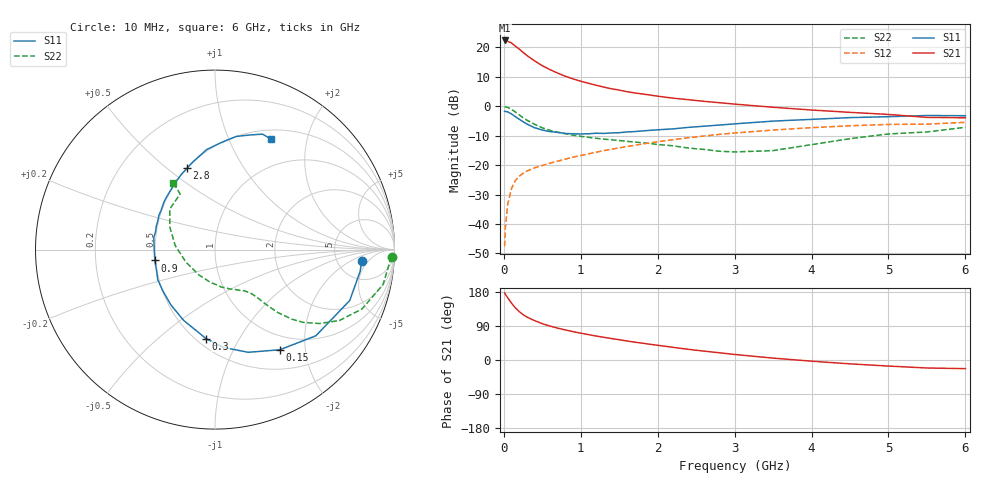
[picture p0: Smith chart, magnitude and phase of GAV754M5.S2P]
! Infineon Technologies  Discrete & RF Semiconductors
! BF775
! Si NPN RF Bipolar Junction Transistor in SOT23
! VCE = 0.75 V  IC = 4.5 mA
! Common Emitter S-Parameters:  May  1996
# GHz  S  MA  R  50
!  f  S11  S21  S12  S22
! GHz  MAG  ANG  MAG  ANG  MAG  ANG  MAG  ANG
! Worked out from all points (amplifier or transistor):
!   36 points, 10 MHz to 6 GHz, reference 50 ohm
!   highest |S21| = 22.4 dB at 10 MHz (marker M1)
!   |S21| within 3 dB of that: start of sweep to 203.1 MHz
!   unconditionally stable (mu >= 1): 727.6 MHz to end of sweep
!   at 250 MHz: K = 0.49, MSG = 20.5 dB, |S12| = -22.8 dB
!   at 1.4 GHz: K = 1.19, MAG = 7.6 dB, |S12| = -14.6 dB
!   at 6 GHz: K = 1.05, MAG = -0.6 dB, |S12| = -5.5 dB
!   S11 on the Smith chart (normalised r, x): 10 MHz: 8.86, -3.33; 150 MHz: 0.78, -1.55; 300 MHz: 0.56, -0.73; 900 MHz: 0.49, -0.07; 2.8 GHz: 0.50, +0.59; 6 GHz: 0.62, +1.45
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0.01  0.8202 -4.3  13.11 177.0  0.0042 87.2  0.9851 -2.4
0.02  0.8178 -8.5  12.94 173.5  0.0087 84.9  0.9741 -4.7
0.05  0.8025 -20.7  12.72 164.3  0.0216 78.7  0.9565 -11.7
0.1  0.7391 -40.5  11.85 150.0  0.04 69.7  0.8832 -22.0
0.15  0.6647 -57.1  10.49 137.5  0.0548 62.1  0.7977 -29.7
0.2  0.6013 -72.1  9.356 127.8  0.0645 57.0  0.7129 -35.3
0.25  0.5463 -85.3  8.24 119.7  0.0727 53.1  0.6378 -39.5
0.3  0.4981 -95.8  7.28 113.4  0.0791 51.6  0.5793 -42.1
0.4  0.4316 -113.8  5.892 103.9  0.09 49.1  0.494 -45.1
0.5  0.394 -128.7  4.88 95.8  0.0987 48.7  0.4303 -46.7
0.6  0.3704 -141.7  4.183 89.5  0.108 48.9  0.3897 -47.7
0.7  0.3604 -152.1  3.657 84.0  0.1168 49.2  0.3621 -48.4
0.9  0.3406 -169.8  2.913 74.8  0.1366 49.6  0.3229 -50.1
1.1  0.3406 175.4  2.455 67.0  0.1555 50.0  0.2964 -52.7
1.3  0.3456 163.5  2.114 59.9  0.1763 49.7  0.2762 -55.7
1.6  0.3661 148.7  1.766 50.1  0.2071 48.3  0.2536 -61.8
2.2  0.413 126.7  1.372 33.4  0.2707 43.5  0.2128 -79.9
2.8  0.4792 109.0  1.15 19.1  0.3324 36.9  0.1721 -109.2
3.5  0.5595 94.7  0.961 5.0  0.3944 27.7  0.1765 -156.9
4.5  0.6412 79.4  0.788 -10.2  0.4662 14.4  0.2815 153.5
5.5  0.6959 67.6  0.647 -21.1  0.4966 0.9  0.3657 122.1
6  0.69 63.0  0.637 -22.8  0.5332 -2.9  0.4393 122.0
